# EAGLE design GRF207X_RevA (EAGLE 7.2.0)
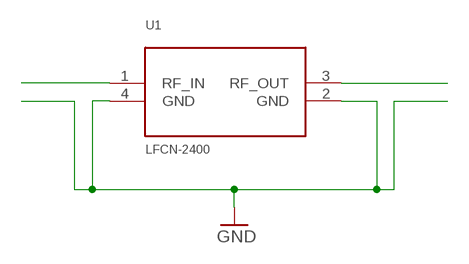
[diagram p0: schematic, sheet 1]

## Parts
U1  LFCN-2400  HFCN-1200  [HFCN-1200]

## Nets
GND: U1.2(GND) U1.4(GND)
N$1: U1.1(RF_IN)
N$4: U1.3(RF_OUT)

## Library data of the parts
U1 = HFCN-1200:HFCN-1200: HFCN-1200+ HFCN-1200 High Pass Filter

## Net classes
0 default: drill 0.152 mm, clearance 0.152 mm
1 RFIN: clearance 0.508 mm to class 0
2 RFOUT: clearance 0.508 mm to class 0
3 POWER: clearance 0.254 mm to class 0
4 FID: clearance 0.178 mm to class 0
5 NC: clearance 0.178 mm to class 0
6 Bypass: clearance 0.203 mm to class 0

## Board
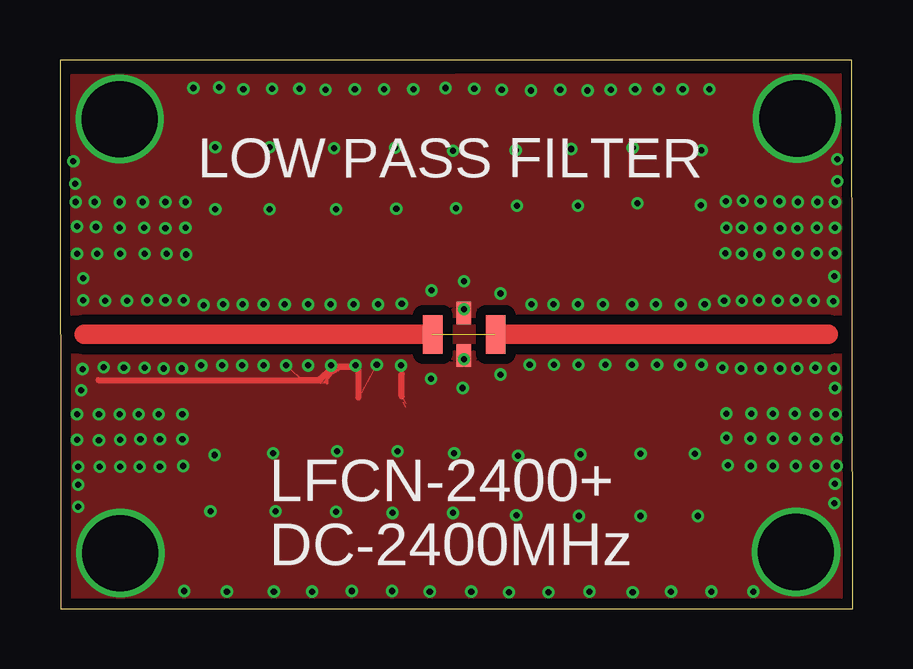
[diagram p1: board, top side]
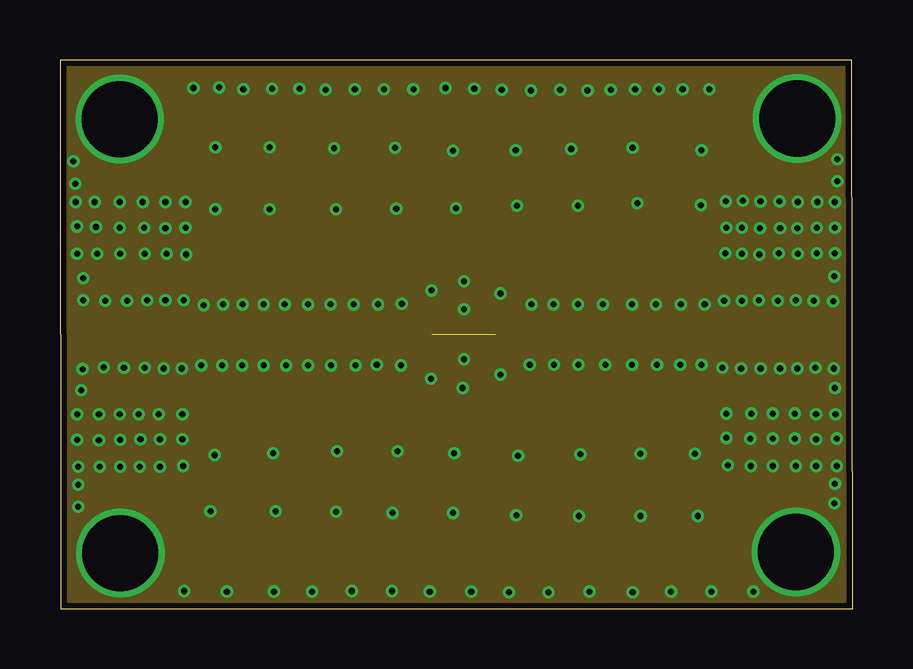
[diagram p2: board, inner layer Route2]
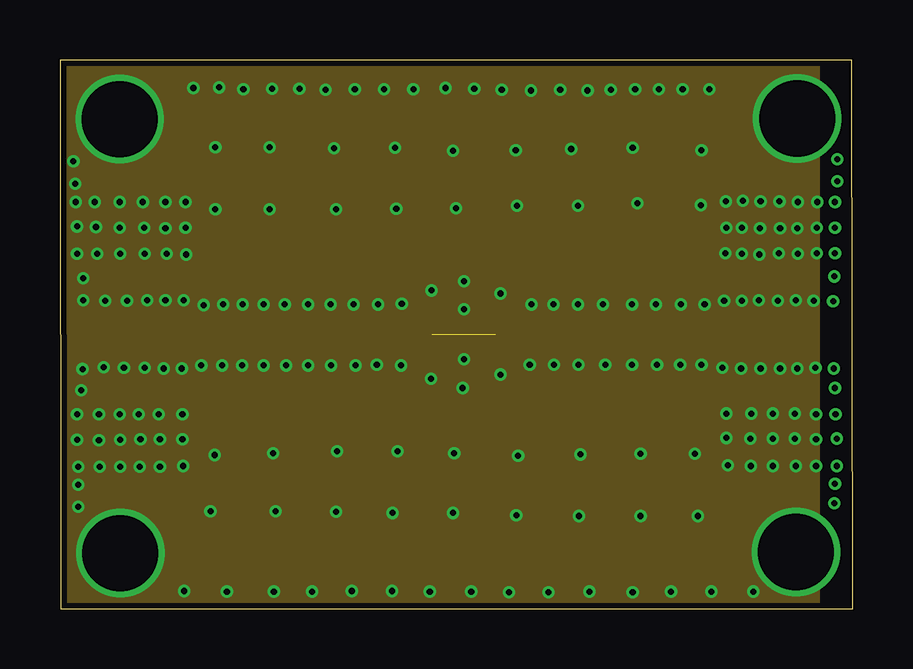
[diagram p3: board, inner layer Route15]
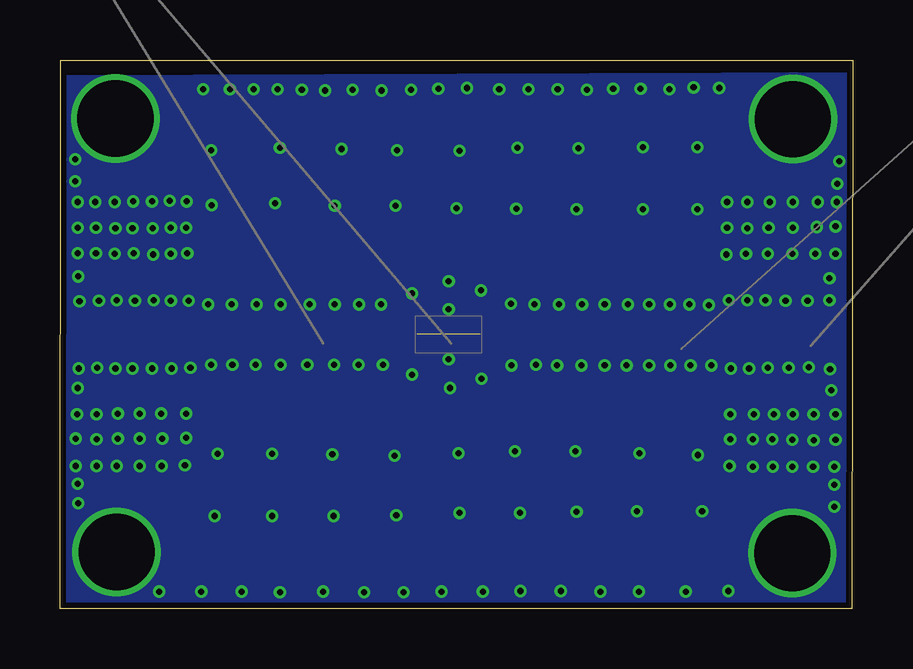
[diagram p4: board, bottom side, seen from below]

Size 33.05 x 22.86 mm. Coordinates in mm from the lower left corner, seen from the top.
Outline: 0.03,0 33.05,0 33.02,22.86 0,22.86 0.03,0
Copper layers (1*2*15*16): Top 0.035559375mm / dielectric 16mil / Route2 0.035559375mm / dielectric 24mil / Route15 0.035559375mm / dielectric 16mil / Bottom 0.035559375mm
Design rules "Eugene_Design_Rules_rev2": minimum track width 1mil, minimum drill 8mil, track to track 6mil, track to pad 4mil, pad to pad 4mil, via to via 4mil, smd to smd 0mil, copper to edge 10mil, drill to drill 8mil, minimum pad ring 5mil, minimum via ring 5mil, stop-mask expansion 0mil, vias tented up to drill 10mil, thermal gap 0mil

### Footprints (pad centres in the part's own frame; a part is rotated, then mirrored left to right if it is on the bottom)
HFCN-1200 = smd 0.813 x 1.6: 1 -0.406,0; 3 2.21,0 | smd 0.61 x 0.94: 2 0.889,-0.889; 4 0.889,0.889

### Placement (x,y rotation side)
U1  15.95,11.43 0 top

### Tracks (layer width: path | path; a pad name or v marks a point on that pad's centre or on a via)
GND  (via drill 0.25, 3.17)
  Top 0.051: 10.74,9.63 11.4,10.21 12.42,10.21 | 10.74,9.63 9.98,9.63 v9.42,10.13 | 10.74,9.63 10.87,9.63 10.79,9.5 | 14.35,8.59 14.3,8.59 14.4,8.38 | v13.21,10.16 12.45,8.79 | 11.13,9.4 10.87,9.37 v11.3,10.13 | 14.25,8.84 14.4,8.56 | 11.15,9.83 11.31,9.78
  Top 0.102: 11.15,9.83 11.13,9.4 | 11.61,9.96 11.31,9.78 11.02,9.42
  Top 0.254: 10.79,9.5 11.46,10.08 12.4,10.08 | 12.45,8.79 12.45,10.13 | 14.25,8.84 14.25,9.78 | 1.6,9.52 10.85,9.52
  other vias: 24.84,12.67 25.88,12.67 31.52,5.94 32.33,8.1 32.26,10.01 22.63,12.67 14.25,12.7 19.66,12.67 25.86,10.16 26.75,10.16 24.89,10.16 23.85,10.16 22.73,10.16 18.36,9.75 16.84,10.39 32.23,12.8 14.22,10.13 8.74,16.64 11.51,16.64 20.6,10.16 32.28,4.39 16.84,13.64 21.62,10.16 18.36,13.13 2.49,16.94 20.57,12.67 28.83,8.13 14.02,16.66 2.51,2.31 2.49,20.4 30.73,20.42 16.84,12.47 0.94,9.98 1.83,10.06 2.67,10.03 3.53,10.03 4.32,10.01 5.08,10.01 1.63,8.1 2.49,8.1 3.28,8.1 4.11,8.1 5.11,8.1 1.63,7.01 4.17,5.92 0.76,5.92 3.63,12.85 5.16,12.85 4.39,12.85 0.71,14.78 2.51,5.92 0.66,16.94 16.08,21.69 13.51,21.64 19.63,21.59 12.29,21.64 0.89,9.09 2.51,7.04 30.68,2.36 15.42,0.71 8.89,6.48 3.33,5.92 17.14,0.71 0.76,5.16 14.73,21.64 0.71,15.93 5.99,12.65 6.81,12.67 7.62,12.67 8.48,12.67 9.37,12.67 8.48,10.13 0.71,7.04 0.71,8.1 5.11,7.06 15.47,9.58 5.56,21.69 12.24,12.67 8.84,21.67 10.34,12.67 13.26,12.67 16.79,9.19 12.32,10.13 5.89,10.13 6.76,10.13 21.59,12.67 23.85,12.67 27.69,12.83 31.5,10.03 26.87,12.67 29.72,7.09 28.4,10.01 27.61,10.03 29.21,10.01 30.02,10.01 30.68,12.85 31.42,12.83 32.31,14.81 32.31,15.88 32.31,16.94 27.79,8.13 27.79,7.11 30.63,7.09 10.34,10.13 7.59,10.13 30.68,5.94 28.8,5.94 32.39,7.09 32.39,5.94 18.41,21.62 15.49,13.26 3.51,15.88 3.45,16.94 22.96,21.62 23.98,21.64 24.97,21.64 28.42,14.78 29.16,14.76 20.85,21.62 19.58,10.16 28.42,12.83 29.13,12.85 29.92,12.83 4.17,7.06 3.35,7.06 30.76,14.78 31.55,14.81 20.37,0.69 28.91,0.71 30.73,10.01 16.43,6.48 27.84,5.97 29.72,8.13 28.78,7.09 31.52,8.1 5.13,5.94 5.18,0.74 1.65,5.92 27.08,21.64 25.96,21.64 6.63,21.72 11.07,21.62 1.88,12.83 2.79,12.83 0.97,12.85 1.45,16.94 0.97,13.77 6.96,0.71 8.92,0.71 10.52,0.71 12.17,0.74 13.84,0.74 0.76,4.24 22.07,0.71 7.65,21.64 9.98,21.67 17.27,21.67 22,21.59 29.97,14.81 23.88,0.69 11.56,6.55 31.52,7.06 30.63,8.13 14.07,6.55 27.15,0.71 25.48,0.71 32.31,5.21 29.72,5.94 18.72,0.69 19.1,6.38 11.28,12.67 5.23,15.88 4.39,16.94 5.23,16.94 0.64,17.7 4.39,15.85 2.49,15.88 4.45,14.78 3.53,14.78 1.5,15.9 2.51,14.78 1.55,14.78 5.26,14.76 0.56,18.64 8.74,19.23 11.43,19.18 13.97,19.2 16.38,19.08 19,19.1 21.31,19.15 23.88,19.2 26.75,19.1 24.08,16.89 21.59,16.79 19.05,16.79 16.51,16.69 27.74,14.81 32.31,9.19 32.28,13.84 31.55,15.88 30.73,15.85 30.02,15.85 29.18,15.85 28.42,15.88 27.79,15.88 31.57,16.94 30.76,16.94 30,16.97 29.21,16.97 28.47,16.99 27.76,16.97 32.41,17.81 32.41,18.72 21.69,6.43 24.21,6.45 26.72,16.81 6.48,19.23 6.48,16.64 6.45,6.4 26.47,6.45 26.59,3.86 24.21,3.86 21.64,3.86 19.02,3.89 16.38,3.99 13.87,3.99 11.51,4.04 8.99,4.06 6.27,4.06
  pour Bottom: -0.03,22.1 32.99,21.97 32.99,-0.23 -0.03,-0.25
  pour Top (isolate 0.432): -0.03,22.07 32.99,22.12 32.99,-0.23 -0.03,-0.25
  pour Route2: -4.34,27.05 32.99,27.05 32.99,-7.75 -4.34,-7.75
  pour Route15: -4.85,27.81 31.47,27.81 31.47,-8.76 -4.85,-8.76
  pour Top: 26.04,9.65 25.98,9.65 25.83,9.5 25.83,8.86 25.96,8.74 26.7,8.74 26.72,8.76 26.72,9.37 26.7,9.4
N$4  (1 unrouted)
  Top 0.813: U1.3 32.03,11.43 | 1.02,11.43 15.52,11.43

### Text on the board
Route2: Metal Layer 2 Ground Plane
Route15: Metal Layer 3 Ground Plane
tNames: LOW PASS FILTER | LFCN-2400+ / DC-2400MHz
Drills: Drill Drawing
bDocu: REV | Description | Date | 1 | Initial release | 05/04/2017 | Required files: / See Readme | Note A: | Note A: | Specifications: / All units are in inches unless otherwise specified. / 1. Materials / Beginning foil thickness 1/2oz min. but shall meet the minimum requirements below: / Layer 1 - Top Layer, 1 oz copper, 0.0014 / Dielectric - Rogers 4003, 0.016 +/- 0.0006 / Layer 2 - Ground Plane, 1 oz copper, 0.0014 / Dielectric - Fr4, (adjust this layer to meet thickness target) / Layer 3 - Ground Plane, 1 oz copper, 0.0014 / Dielectric - Rogers 4003, 0.016 +/- 0.0006 / Layer 4 - Bottom Layer, 1 oz copper, 0.0014 / / Total Board Thickness = 0.062 +/- 0.005 including top and bottom soldermask. / / 2. Hole Plating / Copper plate 0.0010/0.0015 thick in Thru Hole Vias (Approx. 0.0015 on surface). / / 3. Finish / ENIG / Thickness 3-8 micro inches. / Solder Mask / Liquid Photo Imagable (LPI) Solder Mask Over Bare Copper (SMOBC) on Both Sides of PCB. / Color: Red or Approved Equal. / Silkscreen: White Non-Conductive Epoxy Ink. / Supplier ID and Lot Number shall be noted on bottom silkscreen. / 4. Tolerances / Overall board dimension tolerance +/- 0.010. / Hole Diameter >= 0.100 +/- 0.005. / Hole Diameter < 0.100 +/- 0.003. / Layer to layer registration should be +/- 0.001. / All holes shall be located within hole to pad tangency. / 5. Traces / Conductors indicated as Note A shall be 0.030 +/- 0.001 wide and have a coplanar / ground spacing of 0.020 +/- 0.001 Manufacturer shall test for lines indicated to be / 50 Ohm +/- 10% and may adjust the width as needed. / Minimum conductor width is 0.006 +/- 0.001. / Minimum conductor to conductor spacing is 0.006. / TDR coupon required to be delivered with boards. / The controlled impedance on layer 1 shall be 50 Ohms +/- 10%. | SIZE | DOCUMENT NO. | REV | Dimensions are in inches unless / otherwise specified. | A | GRF207X | Date: | Drawn By: Eugenio M. Proenza | SCALE NONE | Sheet 1 of 1 | 05/04/2017
DrillLegend: LAYER-STACK
DrillLegend_01-16: 01-16

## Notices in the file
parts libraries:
SparkFun-Aesthetics: Licensing: Creative Commons ShareAlike 4.0 International - https://creativecommons.org/licenses/by-sa/4.0
